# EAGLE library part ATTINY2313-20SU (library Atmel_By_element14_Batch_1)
8-bit Microcontroller with 2K Bytes In-System Programmable Flash
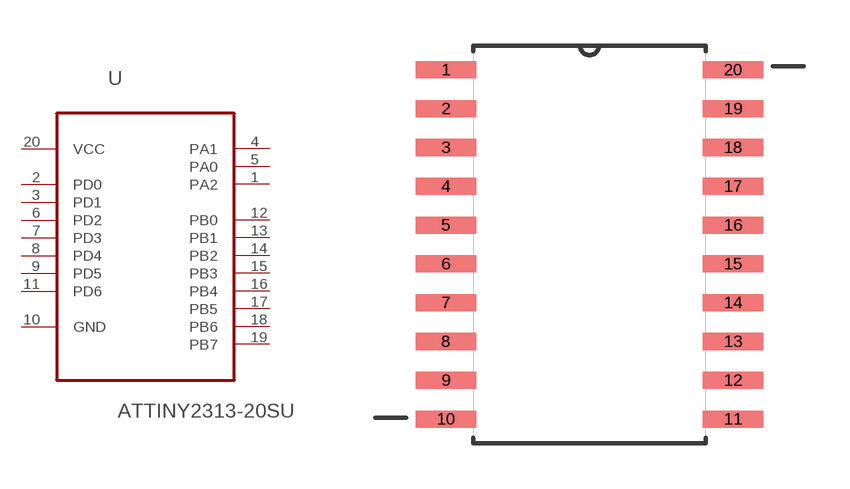
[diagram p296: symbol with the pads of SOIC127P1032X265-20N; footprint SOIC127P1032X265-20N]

Designator prefix U

## ATTINY2313-20SU (MPN: ATTINY2313-20SU; OC_FARNELL: 9171606; OC_NEWARK: 96K6526; PACKAGE: SOIC-20; SUPPLIER: Atmel)  [SOIC127P1032X265-20N]
1  PA2
2  PD0
3  PD1
4  PA1
5  PA0
6  PD2
7  PD3
8  PD4
9  PD5
10  GND  pas
11  PD6
12  PB0
13  PB1
14  PB2
15  PB3
16  PB4
17  PB5
18  PB6
19  PB7
20  VCC  pwr

## Footprint SOIC127P1032X265-20N (pad centres in mm)
smd 1.981 x 0.559: 1 -4.699,5.715; 2 -4.699,4.445; 3 -4.699,3.175; 4 -4.699,1.905; 5 -4.699,0.635; 6 -4.699,-0.635; 7 -4.699,-1.905; 8 -4.699,-3.175; 9 -4.699,-4.445; 10 -4.699,-5.715; 11 4.699,-5.715; 12 4.699,-4.445; 13 4.699,-3.175; 14 4.699,-1.905; 15 4.699,-0.635; 16 4.699,0.635; 17 4.699,1.905; 18 4.699,3.175; 19 4.699,4.445; 20 4.699,5.715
